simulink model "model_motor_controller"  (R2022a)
settings: Solver=VariableStepAuto  StartTime=0.0  StopTime=10  RelTol=1e-3
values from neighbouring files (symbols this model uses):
  B = 1e-5    (= 1e-05)    [motor_controller.m]
  J = 1e-4    (= 0.0001)    [motor_controller.m]
  k = 2e-2    (= 0.02)    [motor_controller.m]
  Ka_i = 1 / Kp_i    (= 0.2)    [motor_controller.m]
  Ka_s = 1 / Kp_s    (= 0.2)    [motor_controller.m]
  Ki_i = Kp_i * Ra / La    (= 1000)    [motor_controller.m]
  Ki_s = J * omega_cs^2 / (5 * k)    (= 1000)    [motor_controller.m]
  Kp_i = La * omega_cc    (= 5)    [motor_controller.m]
  Kp_p = 2.5    [motor_controller.m]
  Kp_s = J * omega_cs / k    (= 5)    [motor_controller.m]
  La = 1e-3    (= 0.001)    [motor_controller.m]
  Ra = 0.2    [motor_controller.m]

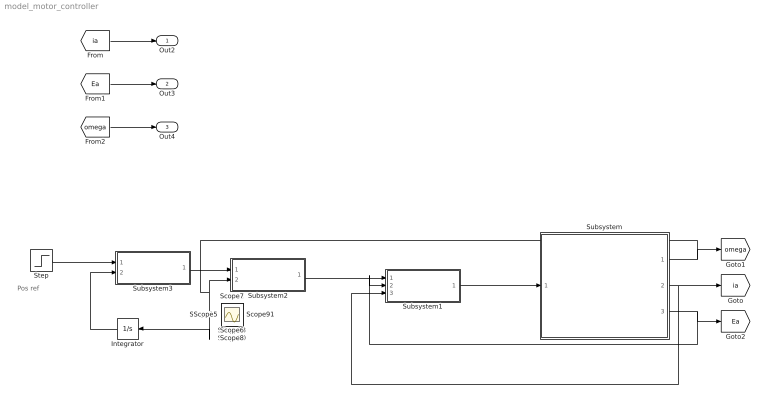
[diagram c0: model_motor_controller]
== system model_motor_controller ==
  note: Pos ref
  Integrator : Integrator
  Step : Step  After=180  SampleTime=0
  Subsystem : Subsystem  Tag=PMDC  Description=PMDC
  Subsystem1 : Subsystem  Description=PI controller
  Subsystem2 : Subsystem  Description=PI controller
  Subsystem3 : Subsystem  Description=PI controller
  Out2 : Outport
  Out3 : Outport  Port=2
  Out4 : Outport  Port=3
  Scope{,1..13} (14 alike) : Scope
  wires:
  Subsystem/1(Out1) -> Integrator/1, Subsystem2/2(In3), [omega]
  [ia] -> Out2/1
  [Ea] -> Out3/1
  [omega] -> Out4/1
  Subsystem/3(Out3) -> Subsystem1/2(In2), [Ea]
  Subsystem/2(Out2) -> [ia], Subsystem1/3(In3)
  Subsystem1/1(Out1) -> Subsystem/1(In1)
  Subsystem2/1(Out1) -> Subsystem1/1(In1)
  Step/1 -> Subsystem3/1(In1)
  Integrator/1 -> Subsystem3/2(In3)
  Subsystem3/1(Out1) -> Subsystem2/1(In1)

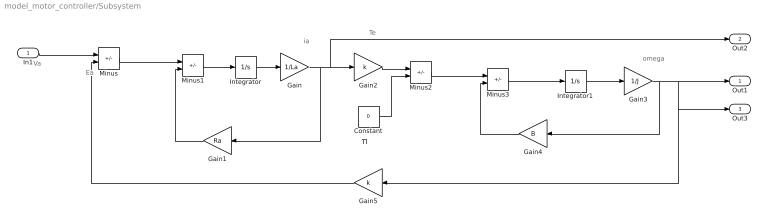
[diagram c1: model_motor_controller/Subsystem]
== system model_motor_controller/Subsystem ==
  note: Ea
  note: Va
  note: Te
  note: Tl
  note: omega
  note: ia
  In1 : Inport
  Constant : Constant  Value=0
  Gain : Gain  Gain=1/La
  Gain1 : Gain  Gain=Ra
  Gain2 : Gain  Gain=k
  Gain3 : Gain  Gain=1/J
  Gain4 : Gain  Gain=B
  Gain5 : Gain  Gain=k
  Integrator : Integrator
  Integrator1 : Integrator
  Minus{,1..3} (4 alike) : Sum  Inputs=+-
  Out1 : Outport
  Out2 : Outport  Port=2
  Out3 : Outport  Port=3
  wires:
  Minus/1 -> Minus1/1
  Gain1/1 -> Minus1/2
  Minus1/1 -> Integrator/1
  Integrator/1 -> Gain/1
  Gain/1 -> Out2/1, Gain2/1, Gain1/1
  Gain2/1 -> Minus2/1
  Constant/1 -> Minus2/2
  Minus2/1 -> Minus3/1
  Minus3/1 -> Integrator1/1
  Integrator1/1 -> Gain3/1
  Gain3/1 -> Gain4/1, Gain5/1, Out3/1, Out1/1
  Gain4/1 -> Minus3/2
  In1/1 -> Minus/1
  Gain5/1 -> Minus/2

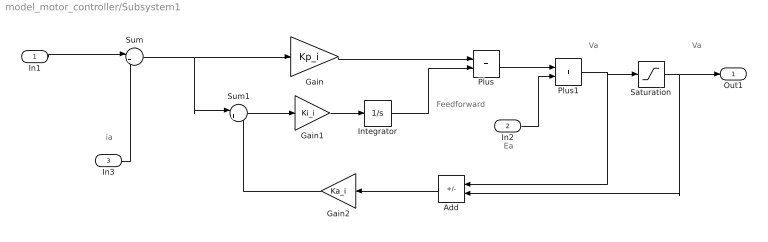
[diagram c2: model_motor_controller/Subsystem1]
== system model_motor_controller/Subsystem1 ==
  note: ia
  note: Ea
  note: Feedforward
  note: Va
  note: Va
  In1 : Inport
  In2 : Inport  Port=2
  In3 : Inport  Port=3
  Add : Sum  Inputs=+-
  Gain : Gain  Gain=Kp_i
  Gain1 : Gain  Gain=Ki_i
  Gain2 : Gain  Gain=Ka_i
  Integrator : Integrator
  Plus : Sum
  Plus1 : Sum
  Saturation : Saturate  UpperLimit=12  LowerLimit=-12
  Sum : Sum  Inputs=|+-
  Sum1 : Sum  Inputs=|+-
  Out1 : Outport
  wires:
  Gain1/1 -> Integrator/1
  Sum/1 -> Sum1/1, Gain/1
  In1/1 -> Sum/1
  Gain/1 -> Plus/1
  Integrator/1 -> Plus/2
  Plus/1 -> Plus1/1
  In2/1 -> Plus1/2
  Plus1/1 -> Add/1, Saturation/1
  Saturation/1 -> Add/2, Out1/1
  Sum1/1 -> Gain1/1
  Gain2/1 -> Sum1/2
  In3/1 -> Sum/2
  Add/1 -> Gain2/1

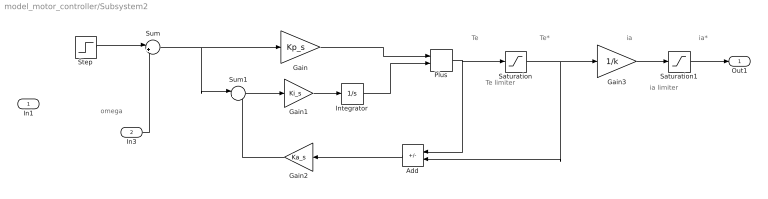
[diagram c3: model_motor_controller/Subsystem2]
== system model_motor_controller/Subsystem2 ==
  note: omega
  note: Te
  note: ia
  note: Te limiter
  note: Te*
  note: ia*
  note: ia limiter
  In1 : Inport
  In3 : Inport  Port=2
  Add : Sum  Inputs=+-
  Gain : Gain  Gain=Kp_s
  Gain1 : Gain  Gain=Ki_s
  Gain2 : Gain  Gain=Ka_s
  Gain3 : Gain  Gain=1/k
  Integrator : Integrator
  Plus : Sum
  Saturation : Saturate  UpperLimit=0.247  LowerLimit=-0.247
  Saturation1 : Saturate  UpperLimit=1  LowerLimit=-1
  Step : Step  After=300  SampleTime=0
  Sum : Sum  Inputs=|+-
  Sum1 : Sum  Inputs=|+-
  Out1 : Outport
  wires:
  Gain1/1 -> Integrator/1
  Sum/1 -> Sum1/1, Gain/1
  Gain/1 -> Plus/1
  Integrator/1 -> Plus/2
  Plus/1 -> Saturation/1, Add/1
  Saturation/1 -> Gain3/1, Add/2
  Sum1/1 -> Gain1/1
  Gain2/1 -> Sum1/2
  In3/1 -> Sum/2
  Add/1 -> Gain2/1
  Gain3/1 -> Saturation1/1
  Saturation1/1 -> Out1/1
  Step/1 -> Sum/1

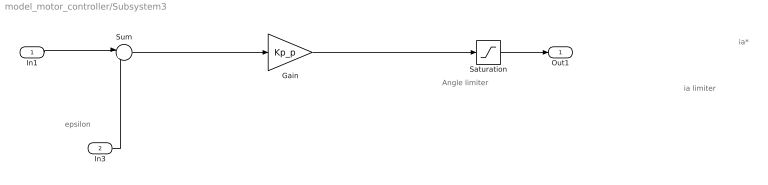
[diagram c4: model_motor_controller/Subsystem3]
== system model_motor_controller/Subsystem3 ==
  note: epsilon
  note: Angle limiter
  note: ia*
  note: ia limiter
  In1 : Inport
  In3 : Inport  Port=2
  Gain : Gain  Gain=Kp_p
  Saturation : Saturate  UpperLimit=360  LowerLimit=0
  Sum : Sum  Inputs=|+-
  Out1 : Outport
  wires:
  Sum/1 -> Gain/1
  In1/1 -> Sum/1
  In3/1 -> Sum/2
  Saturation/1 -> Out1/1
  Gain/1 -> Saturation/1
